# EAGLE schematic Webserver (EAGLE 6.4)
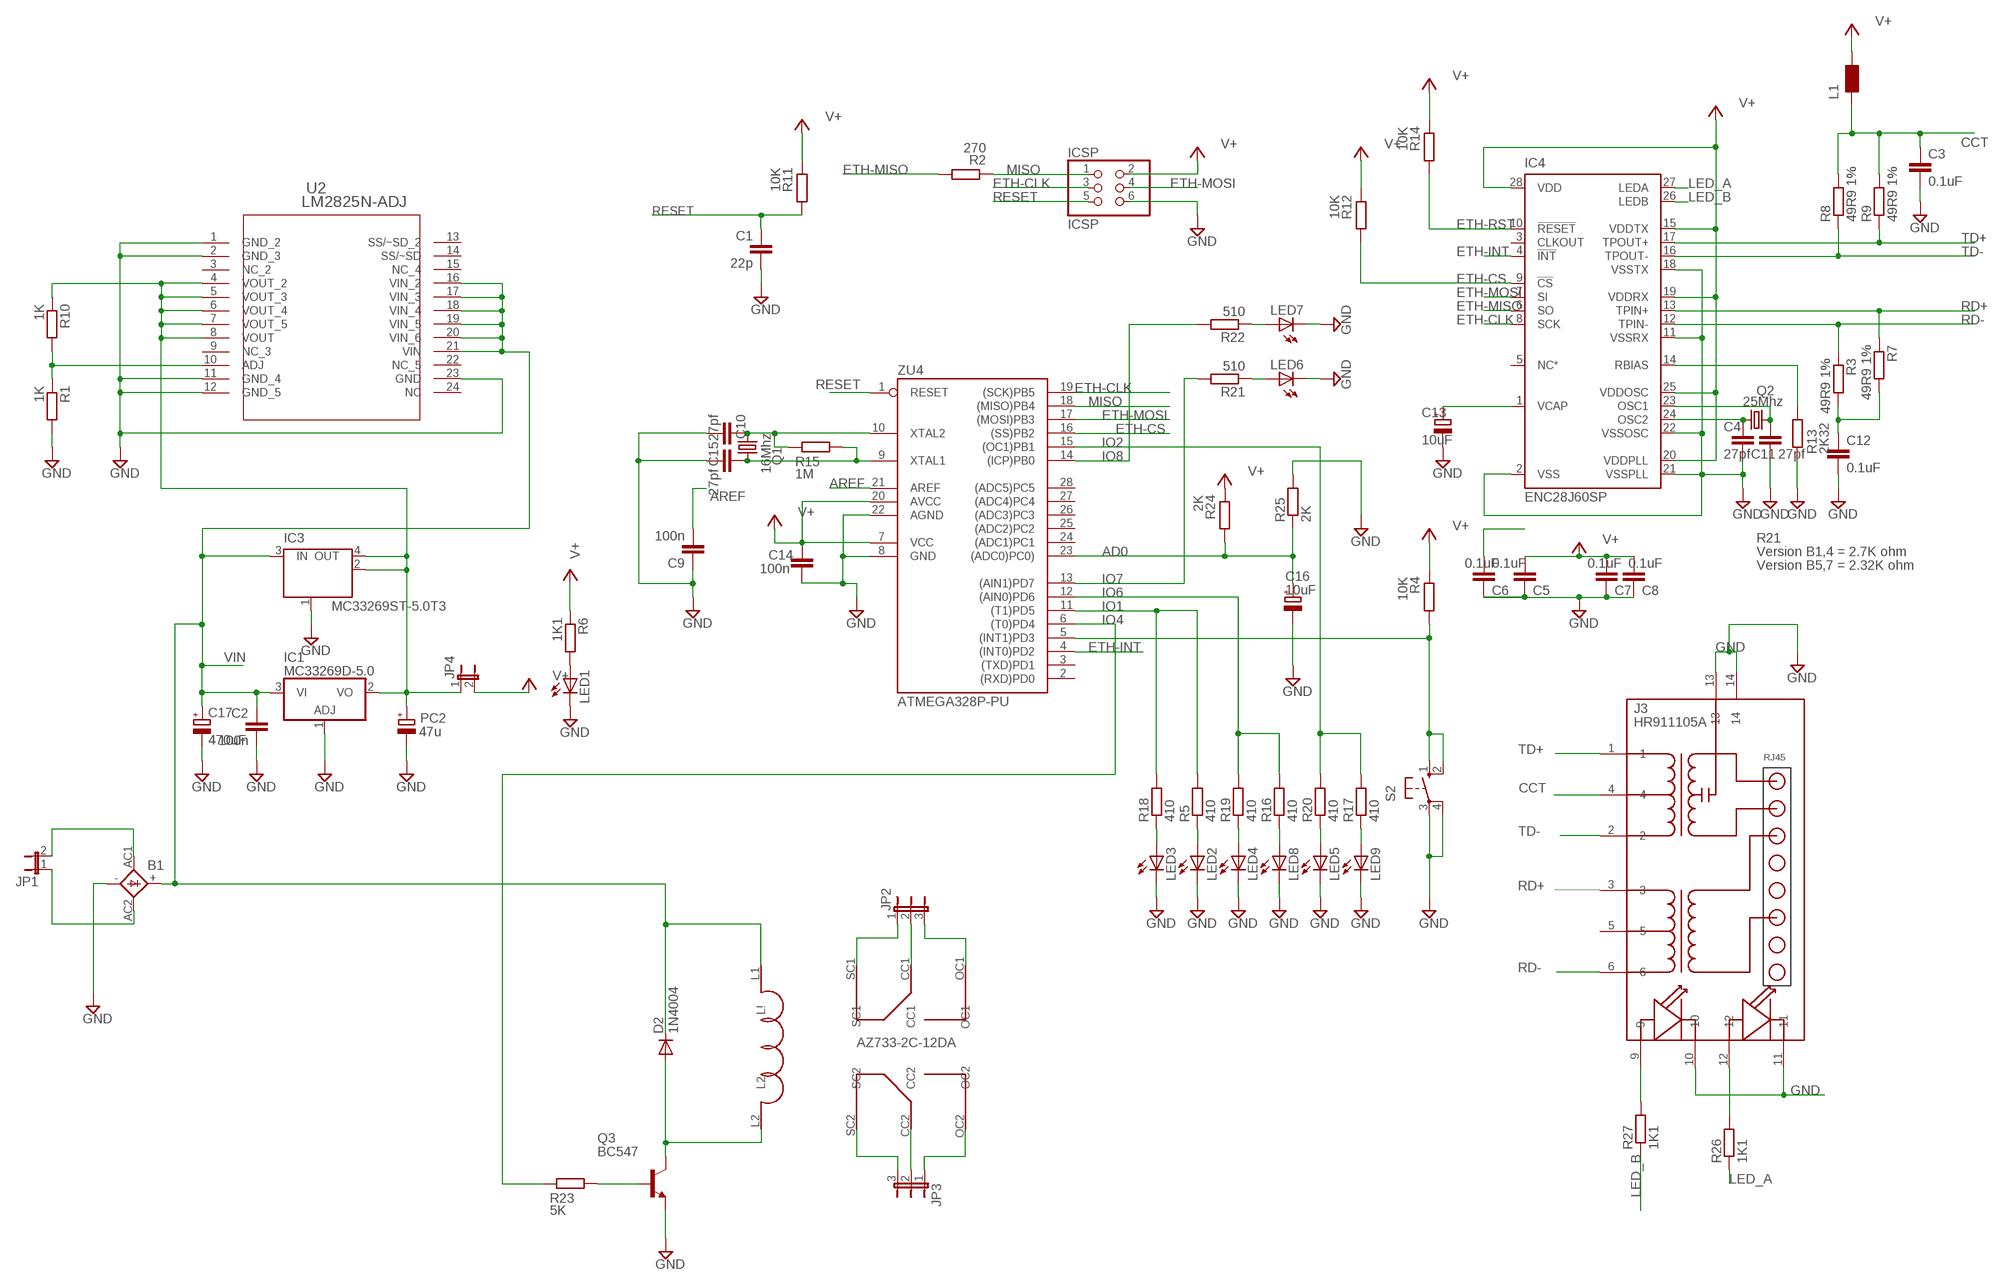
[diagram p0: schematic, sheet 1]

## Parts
B1  2KBB  [2KBB]
C1  22p  C-EU0603-RND  [C0603-ROUND]
C2  100n  C-EU0603-RND  [C0603-ROUND]
C3  0.1uF  C-EUC0805  [C0805]
C4  27pf  C-EUC0805  [C0805]
C5  0.1uF  C-EUC0805  [C0805]
C6  0.1uF  C-EUC0805  [C0805]
C7  0.1uF  C-EUC0805  [C0805]
C8  0.1uF  C-EUC0805  [C0805]
C9  100n  C-EUC0805  [C0805]
C10  27pf  C-EUC0805  [C0805]
C11  27pf  C-EUC0805  [C0805]
C12  0.1uF  C-EUC0805  [C0805]
C13  10uF  CPOL-EUSMCA  [SMC_A]
C14  100n  C-EUC0805  [C0805]
C15  27pf  C-EUC0805  [C0805]
C16  10uF  CPOL-EUSMCA  [SMC_A]
C17  470uF  CPOL-EUE7.5-16  [E7,5-16]
D2  1N4004  [DO41-10]
IC1  MC33269D-5.0  [DPACK]
IC3  MC33269ST-5.0T3  MC33269ST-3.3T3  [SOT223]
IC4  ENC28J60SP  [DIL28-3]
ICSP  ICSP  PINHD-2X3  [2X03]
J3  HR911105A  [HR911105A]
JP1  JP1E  [JP1]
JP2  JP2E  [JP2]
JP3  JP2E  [JP2]
JP4  JP1E  [JP1]
L1  WE-KIL_0805  [WE-KI_0805_B]
LED1  LED5MM  [LED5MM]
LED2  LED5MM  [LED5MM]
LED3  LED5MM  [LED5MM]
LED4  LED5MM  [LED5MM]
LED5  LED5MM  [LED5MM]
LED6  LED5MM  [LED5MM]
LED7  LED5MM  [LED5MM]
LED8  LED5MM  [LED5MM]
LED9  LED5MM  [LED5MM]
PC2  47u  CPOL-EUD  [PANASONIC_D]
Q1  16Mhz  CRYSTALHC49S  [HC49/S]
Q2  25Mhz  CRYSTALHC49S  [HC49/S]
Q3  BC547  [TO92]
R1  1K  R-EU_R2012  [R2012]
R2  270  R-EU_R0805  [R0805]
R3  49R9 1%  R-EU_R0805  [R0805]
R4  10K  R-EU_R0805  [R0805]
R5  410  R-EU_R0805  [R0805]
R6  1K1  R-EU_R0805  [R0805]
R7  49R9 1%  R-EU_R0805  [R0805]
R8  49R9 1%  R-EU_R0805  [R0805]
R9  49R9 1%  R-EU_R0805  [R0805]
R10  1K  R-EU_R2012  [R2012]
R11  10K  R-EU_R0805  [R0805]
R12  10K  R-EU_R0805  [R0805]
R13  2K32  R-EU_R0805  [R0805]
R14  10K  R-EU_R0805  [R0805]
R15  1M  R-EU_R0805  [R0805]
R16  410  R-EU_R0805  [R0805]
R17  410  R-EU_R0805  [R0805]
R18  410  R-EU_R0805  [R0805]
R19  410  R-EU_R0805  [R0805]
R20  410  R-EU_R0805  [R0805]
R21  510  R-EU_R0805  [R0805]
R22  510  R-EU_R0805  [R0805]
R23  5K  R-EU_R0805  [R0805]
R24  2K  R-EU_R0805  [R0805]
R25  2K  R-EU_0204/7  [0204/7]
R26  1K1  R-EU_R0805  [R0805]
R27  1K1  R-EU_R0805  [R0805]
S2  10-XX  [B3F-10XX]
U2  LM2825N-ADJ  [NA24F]
U$1  AZ733_2C_12DA  [AZ733_2C_12DA]
ZU4  ATMEGA328P-PU  [DIL28-3]

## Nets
AD0: C16.+ R24.2 R25.1 ZU4.23((ADC0)PC0))
AREF [aref]: C9.2 ZU4.21(AREF)
CCT: C3.1 J3.4 L1.2 R8.2 R9.2
ETH-CLK: IC4.8(SCK) ICSP.3 ZU4.19((SCK)PB5)
ETH-CS: IC4.9(!CS) R12.2 ZU4.16((SS)PB2)
ETH-INT: IC4.4(!INT) ZU4.4((INT0)PD2)
ETH-MISO: IC4.6(SO) R2.2
ETH-MOSI: IC4.7(SI) ICSP.4 ZU4.17((MOSI)PB3)
ETH-RST: IC4.10(!RESET) R14.2
GND: B1.- C1.2 C2.2 C3.2 C4.2 C5.2 C6.2 C7.2 C8.2 C9.1 C10.2 C11.2 C12.2 C13.- C14.1 C15.2 C16.- C17.- IC1.1(ADJ) IC3.1(GND/ADJ) IC4.2(VSS) IC4.11(VSSRX) IC4.18(VSSTX) IC4.21(VSSPLL) IC4.22(VSSOSC) ICSP.6 J3.10 J3.11 J3.13 J3.14 LED1.K(C) LED2.K(C) LED3.K(C) LED4.K(C) LED5.K(C) LED6.K(C) LED7.K(C) LED8.K(C) LED9.K(C) PC2.- Q3.1(E) R1.2 R13.1 R25.2 S2.3(P) S2.4(P1) U2.1(GND_2) U2.2(GND_3) U2.11(GND_4) U2.12(GND_5) U2.23(GND) ZU4.8(GND) ZU4.22(AGND)
IO1: R5.2 R18.2 ZU4.11((T1)PD5)
IO2: R17.2 R20.2 ZU4.15((OC1)PB1)
IO4: R23.1 ZU4.6((T0)PD4)
IO6: R16.2 R19.2 ZU4.12((AIN0)PD6)
IO7: R21.2 ZU4.13((AIN1)PD7)
IO8: R22.2 ZU4.14((ICP)PB0)
LED_A: IC4.27(LEDA) R26.1
LED_B: IC4.26(LEDB) R27.1
LED_STATUS: J3.12 R26.2
MISO: ICSP.1 R2.1 ZU4.18((MISO)PB4)
N$1: LED2.A R5.1
N$2: C4.1 IC4.24(OSC2) Q2.1
N$3: C11.1 IC4.23(OSC1) Q2.2
N$4: C12.1 R3.2 R7.2
N$5: IC4.14(RBIAS) R13.2
N$6: C15.1 Q1.2 R15.2 ZU4.9(XTAL1)
N$7: LED1.A R6.2
N$8: C13.+ IC4.1(VCAP)
N$9: LED8.A R16.1
N$10: LED3.A R18.1
N$11: LED4.A R19.1
N$12: LED5.A R20.1
N$13: Q3.2(B) R23.2
N$14: JP3.3 U$1.SC2
N$15: LED6.A R21.1
N$16: LED7.A R22.1
N$17: D2.A Q3.3(C) U$1.L2
N$18: JP3.2 U$1.CC2
N$19: J3.9 R27.2
N$20: JP3.1 U$1.OC2
N$21: R1.1 R10.2 U2.10(ADJ)
N$22: B1.AC2 JP1.1
N$23: B1.AC1 JP1.2
N$24: JP2.2 U$1.CC1
N$25: JP2.1 U$1.SC1
N$26: JP2.3 U$1.OC1
N$27: R4.2 S2.1(S) S2.2(S1) ZU4.5((INT1)PD3)
N$29: LED9.A R17.1
N$30: C6.1 IC1.2(VO) IC3.2(OUT) IC3.4(OUT) JP4.1 PC2.+ R10.1 U2.4(VOUT_2) U2.5(VOUT_3) U2.6(VOUT_4) U2.7(VOUT_5) U2.8(VOUT)
RD+: IC4.13(TPIN+) J3.3 R7.1
RD-: IC4.12(TPIN-) J3.6 R3.1
RESET: C1.1 ICSP.5 R11.2 ZU4.1(RESET)
TD+: IC4.17(TPOUT+) J3.1 R9.1
TD-: IC4.16(TPOUT-) J3.2 R8.1
V+: C5.1 C7.1 C8.1 C14.2 IC4.15(VDDTX) IC4.19(VDDRX) IC4.20(VDDPLL) IC4.25(VDDOSC) IC4.28(VDD) ICSP.2 JP4.2 L1.1 R4.1 R6.1 R11.1 R12.1 R14.1 R24.1 ZU4.7(VCC) ZU4.20(AVCC)
VIN: B1.+ C2.1 C17.+ D2.C IC1.3(VI) IC3.3(IN) U2.16(VIN_2) U2.17(VIN_3) U2.18(VIN_4) U2.19(VIN_5) U2.20(VIN_6) U2.21(VIN) U$1.L1(L!)
XTAL2: C10.1 Q1.1 R15.1 ZU4.10(XTAL2)
Unconnected: IC4.3(CLKOUT) IC4.5(NC*) J3.5 U2.3(NC_2) U2.9(NC_3) U2.13(SS/~SD_2) U2.14(SS/~SD) U2.15(NC_4) U2.22(NC_5) U2.24(NC) ZU4.2((RXD)PD0) ZU4.3((TXD)PD1) ZU4.24((ADC1)PC1) ZU4.25((ADC2)PC2) ZU4.26((ADC3)PC3) ZU4.27((ADC4)PC4) ZU4.28((ADC5)PC5)

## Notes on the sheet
- R21
- Version B1,4 = 2.7K ohm
- Version B5,7 = 2.32K ohm

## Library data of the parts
B1 = rectifier:2KBB: RECTIFIER grid 3 x 5 mm
C1 C2 = SmartPrj:C-EU: CAPACITOR, European symbol
C3-C12 C14 C15 = rcl:C-EU: CAPACITOR, European symbol
C13 C16 C17 PC2 = rcl:CPOL-EU: POLARIZED CAPACITOR, European symbol
D2 = diode:1N4004: DIODE
IC1 = linear:MC33269?*: Adjustable Output Low Dropout Voltage Regulator 800 mA Source: http://www.onsemi.com/pub/Collateral/MC33269-D.PDF
IC3 = linear:MC33269ST*: Adjustable Output Low Dropout Voltage Regulator 800 mA Source: http://www.onsemi.com/pub/Collateral/MC33269-D.PDF
IC4 = microchip:ENC28J60: Stand-Alone Ethernet Controller with SPI Interface Source: http://ww1.microchip.com/downloads/en/DeviceDoc/39662c.pdf; MF: MICROCHIP; MPN: ENC28J60/SP; OC_FARNELL: 1084619; OC_NEWARK: 96K3661
ICSP = pinhead:PINHD-2X3: PIN HEADER
J3 = CONNECTER:HR911105A
JP1 JP4 = jumper:JP1E: JUMPER
JP2 JP3 = jumper:JP2E: JUMPER
L1 = wuerth-elektronik:WE-KIL: SMD Wire Wound Ceramic Inductor WE-KIL
LED1-LED9 = led:LED: LED
Q1 Q2 = crystal:CRYSTAL: CRYSTAL; OC_FARNELL: 1667008; OC_NEWARK: unknown
Q3 = transistor-npn:BC547*: NPN Transistor
R1-R27 = rcl:R-EU_: RESISTOR, European symbol
S2 = switch-omron:10-XX: OMRON SWITCH; MPN: B3F-1000; OC_FARNELL: 176432; OC_NEWARK: 36M3542
U2 = LM2825N_ADJ:LM2825N-ADJ; BASE_PN: LM2825; COMPTYPE: Switcher; MANUFACTURER_PART_NUMBER: LM2825N-ADJ; SYMBOL: NameLM2825N-ADJ; TYPE: LM2825N-ADJ; VENDOR: National; VERSION: 05/02/2007
U$1 = AZ733:AZ733_2C_12DA: American Zettler AZ733 serie relay
ZU4 = SmartPrj:ATMEGA328P-: MICROCONTROLLER 4 Kbytes FLASH 128 bytes SRAM 256 bytes EEPROM UART 6-channel 10 bit ADC

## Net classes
0 default: width 0.152 mm, drill 0.305 mm, clearance 0.152 mm
2 gnd: width 0.305 mm, drill 0.559 mm, clearance 0.254 mm
3 usbvcc: width 0.508 mm, drill 0.61 mm, clearance 0.254 mm
4 aref: width 0.406 mm, drill 0.61 mm, clearance 0.254 mm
